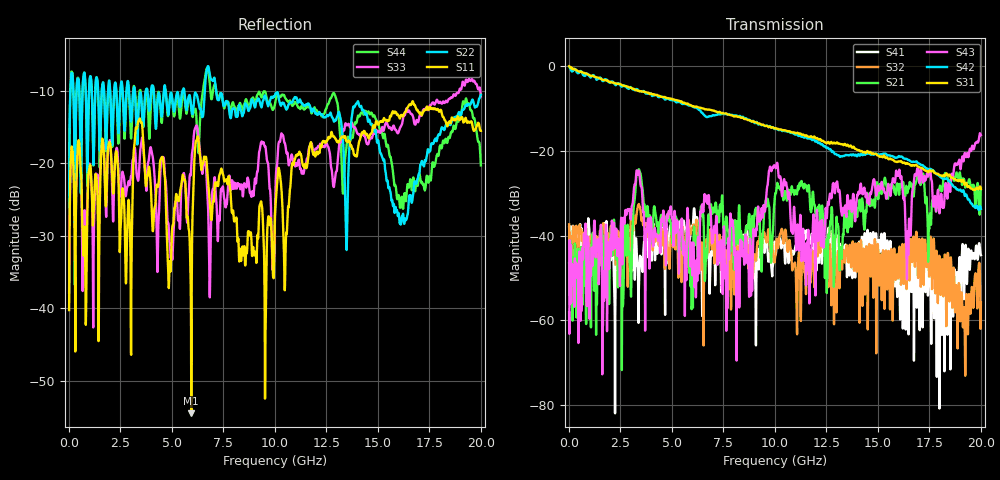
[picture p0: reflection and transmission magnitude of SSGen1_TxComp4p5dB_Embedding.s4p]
! C:\Users\lab_ccd01\Downloads\USBIF_ISI1_4p5dB_at_2p5GHz.s4p
! Sun Feb 23 11:44:49 2025
!!Measured using Teledyne LeCroy WavePulser LCRY4802N20219
!MixedMode
!DutToConverterPinDefinitions,+1,-1,+2,-2
!UserPortDefinitions,D1,C1,D2,C2
! freq S11 S12 S13 S14
! S21 S22 S23 S24
! S31 S32 S33 S34
! S41 S42 S43 S44
# GHz S dB R 50.00
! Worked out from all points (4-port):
!   2000 points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, 10 MHz to 20 GHz, reference 50 ohm
!   strongest paths, dB at 10 MHz, 5.01 GHz, 10.01 GHz, 15.01 GHz, 20 GHz:
!     S31: 0.0, -7.9, -14.7, -21.1, -29.0
!     S42: -0.1, -8.1, -14.8, -20.8, -33.7
!     S43: -58.1, -35.9, -23.9, -28.3, -16.3
!     S21: -46.5, -40.8, -30.4, -31.4, -28.8
!     S32: -37.4, -39.6, -45.2, -42.8, -55.7
!     S41: -38.0, -40.1, -42.6, -43.1, -44.6
!   lowest |S11| = -54.5 dB at 5.94 GHz (marker M1), VSWR 1.00, Z = 49.8 - j0.0521 ohm
!   |S11| at or under -10 dB: start of sweep to end of sweep
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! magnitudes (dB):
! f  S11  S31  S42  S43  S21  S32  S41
! 10 MHz  -40.2  0.0  -0.1  -58.1  -46.5  -37.4  -38.0
! 2.57 GHz  -25.0  -4.5  -4.8  -39.4  -71.7  -41.3  -40.9
! 3.38 GHz  -14.2  -5.9  -5.8  -24.8  -24.5  -32.8  -60.6
! 5.94 GHz  -54.5  -9.3  -9.4  -41.9  -49.5  -38.8  -37.7
! 10.02 GHz  -26.1  -14.7  -14.8  -24.0  -30.1  -44.9  -43.4
! 16.44 GHz  -12.3  -23.0  -22.1  -39.0  -29.7  -41.3  -46.6
! 20 GHz  -15.5  -29.0  -33.7  -16.3  -28.8  -55.7  -44.6
